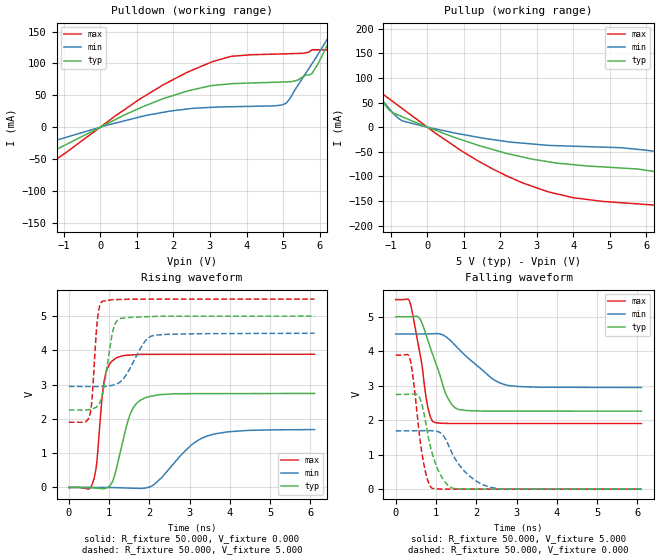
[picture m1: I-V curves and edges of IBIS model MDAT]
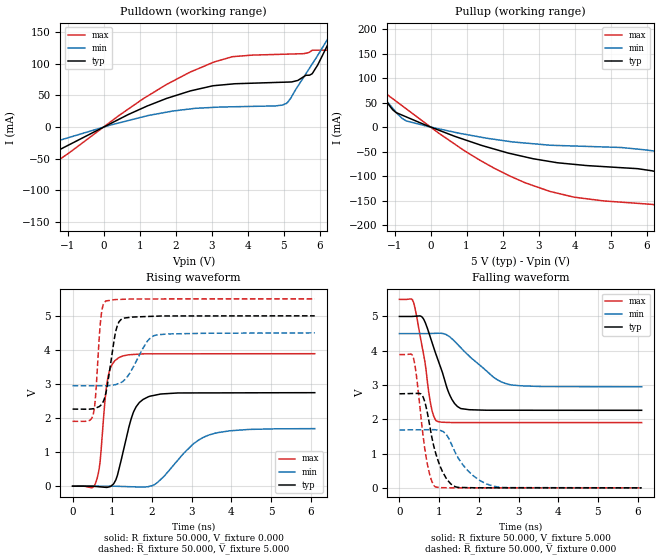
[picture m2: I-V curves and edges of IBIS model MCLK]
|Texas Instruments Incorporated
|1-Bit, 10MHz, 2nd-Order, Isolated Delta-Sigma Modulator
| Marketing part#  Voltage Range   Package-type   #pins
|AMC1203BDUB   4.5 to 5.5   SO-8, Gull-Wing   8
|AMC1203BDUBG4   4.5 to 5.5   SO-8, Gull-Wing   8
|AMC1203BDUBR   4.5 to 5.5   SO-8, Gull-Wing   8
|AMC1203BDUBRG4   4.5 to 5.5   SO-8, Gull-Wing   8
|AMC1203DUB   4.5 to 5.5   SO-8, Gull-Wing   8
|AMC1203DUBG4   4.5 to 5.5   SO-8, Gull-Wing   8
|AMC1203DUBR   4.5 to 5.5   SO-8, Gull-Wing   8
|AMC1203DUBRG4   4.5 to 5.5   SO-8, Gull-Wing   8
|AMC1203BDW   4.5 to 5.5   SO-16   16
|AMC1203BDWR   4.5 to 5.5   SO-16   16
|AMC1203DW   4.5 to 5.5   SO-16   16
|AMC1203DWR   4.5 to 5.5   SO-16   16
|AMC1203BPSA   4.5 to 5.5   SO-8   8
|AMC1203BPSAR   4.5 to 5.5   SO-8   8
|AMC1203PSA   4.5 to 5.5   SO-8   8
|AMC1203PSAR   4.5 to 5.5   SO-8   8
[IBIS Ver]   4.0
[File name]   amc1203.ibs
[File Rev]   1.0
[Date]   05/062010
[Source]   Texas Instruments Incorporated.
   Analog-eLab, HPA
   12500 TI Blvd
   Dallas, TX -75243
   For Support e-mail: elab_ibis@list.ti.com
[Notes]   Revision History:
   1.0: 05/062010
   - Initial version of the model
   - Initial Model generated from simulations in TISPICED
   - Specified temperature range = -40C to 105C. Device power
   dissipation is 110mW. Maximum theta jc (SO-8) = 164 C/W. IBIS
   test maximum temperature = 125C
   - Model not matched to measurements
   - Ignore warnings related to min and max values of ccomp,
   The device process of this product is CMOS. The ccomp
   values are based on PVT variations as seen in simulations
[Disclaimer]
 This product is designed as an aid for customers of Texas Instruments.
 No warranties, either expressed or implied, with respect to this third
 party software (if any) or with respect to its fitness for any
 particular purpose is claimed by Texas Instruments or the author. The
 software (if any) is provided solely on an "as is" basis. The entire
 risk as to its quality and performance is with the customer
[Copyright] (C) Copyright 2009 Texas Instruments Incorporated.
   All rights reserved.
|   AMC1203DUB - SO-8, Gull-Wing
[Component]   amc1203dub   |SO-8, Gull-Wing
[Manufacturer] TI
[Package]
| variable   typ   min   max
R_pkg  0.067958   0.033850   0.110020
L_pkg  4.035955nH  3.604460nH  4.524820nH
C_pkg  1.196889pF  1.079930pF  1.255480pF
[Pin] signal_name  model_name  R_pin  L_pin C_pin
1   VDD1   TERM   0.04382  4.49301nH  1.20573pF
2   VINP   TERM   0.08107  3.84004nH  1.21759pF
3   VINN   TERM   0.11002  4.52482nH  1.24194pF
4   GND1   TERM   0.03385  3.60446nH  1.12112pF
5   GND2   GND   0.04658  3.76318nH  1.07993pF
6   MDAT   MDAT   0.10060  4.30773nH  1.23091pF
7   MCLK   MCLK   0.08948  4.04013nH  1.22241pF
8   VDD2   POWER   0.03824  3.71427nH  1.25548pF
|   AMC1203PSA - SO-8
[Component]   amc1203pas   |SO-8
[Manufacturer] TI
[Package]
| variable   typ   min   max
R_pkg  0.082216   0.044190   0.126530
L_pkg  1.772578nH  1.469600nH  2.372740nH
C_pkg  0.346504pF  0.239380pF  0.477210pF
[Pin] signal_name  model_name  R_pin  L_pin C_pin
1   VDD1   TERM   0.06196  2.37274nH  0.46610pF
2   VINP   TERM   0.10341  1.72833nH  0.31281pF
3   VINN   TERM   0.12653  1.86934nH  0.25026pF
4   GND1   TERM   0.05629  2.10297nH  0.42922pF
5   GND2   GND   0.06651  1.50308nH  0.29801pF
6   MDAT   MDAT   0.11287  1.66363nH  0.23938pF
7   MCLK   MCLK   0.08597  1.47093nH  0.29904pF
8   VDD2   POWER   0.04419  1.46960nH  0.47721pF
|   AMC1203DW - SO-16
[Component]   amc1203dw   |SO-16
[Manufacturer] TI
[Package]
| variable   typ   min   max
R_pkg  0.038526   0.003610   0.111860
L_pkg  2.946539nH  1.634270nH  4.703810nH
C_pkg  0.921273pF  0.675660pF  1.374930pF
[Pin] signal_name  model_name  R_pin  L_pin C_pin
1   VDD1   TERM   0.04296  4.66236nH  1.26722pF
2   VINP   TERM   0.11186  4.70381nH  1.06049pF
3   VINN   TERM   0.09034  3.30153nH  0.76963pF
4   GND1   TERM   0.00361  1.63447nH  0.70855pF
5   NC   NC   0.00361  1.63427nH  0.70856pF
6   NC   NC   0.00370  1.66394nH  0.68405pF
7   NC   NC   0.00367  1.67094nH  0.67566pF
8   GND1   TERM   0.02804  4.12835nH  1.37395pF
9   GND2   GND   0.03564  4.05816nH  1.37493pF
10   NC   NC   0.09603  3.43032nH  0.78630pF
11   MDAT   MDAT   0.05441  2.62155nH  0.89494pF
12   NC   NC   0.00361  1.63430nH  0.70851pF
13   MCLK   MCLK   0.07390  2.89307nH  0.78596pF
14   VDD2   POWER   0.05191  3.03712nH  0.82076pF
15   NC   NC   0.00565  2.62355nH  0.94964pF
16   GND2   GND   0.00747  3.44688nH  1.17122pF
|   TERM Model
[Model] TERM
Model_type Terminator
C_comp   1e-200   1e-200   1e-200
| variable   typ   min   max
[Voltage Range]   5.0V   4.5V   5.5V
[POWER Clamp Reference]  5.0V   4.5V   5.5V
[GND Clamp Reference]   0.0V   0.0V   0.0V
|Operating Temperature
[Temperature Range]   27   123   -40
| Models and submodels in the file (3): TERM (Terminator), MDAT (Output), MCLK (Output)
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|   MDAT Model
[Model] MDAT
Model_type Output
Polarity   Non-Inverting
Enable   Active-Low
Vmeas = 2.5
Vref = 2.5
Cref = 15pF
Rref = 50
|   typ   min   max
|   MDAT HIGH
C_comp   1.446901E-12   1.464566E-12   1.435600E-012
|   MDAT LOW
|C_comp   3.656083E-13   3.837180E-13   2.354078E-13
|   average
|C_comp   9.062547E-13   7.178000E-02   9.241420E-13
| variable   typ   min   max
[Voltage Range]   5   4.5   5.5
[Temperature Range]   27   125   -40
[Pullup Reference]   5   4.5   5.5
[Pulldown Reference]   0   0   0
[Power Clamp Reference]   5   4.5   5.5
[GND Clamp Reference]   0   0   0
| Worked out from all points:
|   slope of the pulldown table from 0 to 0.75 V, typ, clamps not added: 34.8 ohm
|   slope of the pullup table from 0 to 0.75 V, typ, clamps not added: 35.6 ohm
|   falling waveform, R_fixture 50.000, V_fixture 5.000: 20-80 % time 469ps typ, 877ps min, 292ps max; typ from 5 V to 2.26 V
|   rising waveform, R_fixture 50.000, V_fixture 0.000: 20-80 % time 363ps typ, 832ps min, 180ps max; typ from 0 V to 2.74 V
|   rising waveform, R_fixture 50.000, V_fixture 5.000: 20-80 % time 219ps typ, 442ps min, 122ps max; typ from 2.26 V to 5 V
|   falling waveform, R_fixture 50.000, V_fixture 0.000: 20-80 % time 353ps typ, 595ps min, 245ps max; typ from 2.74 V to 0 V
[Pulldown]
|   Voltage   I(typ)   I(min)   I(max)
-5V       -138.1mA   -85.42mA   -187.7mA
-3.408V   -95.74mA   -58.23mA   -133.2mA
-1.909V   -55.62mA   -32.63mA   -78.2mA
1.207V    33.19mA    17.88mA    48.53mA
3.065V    65.4mA     31.15mA    102.8mA
3.59V     68.14mA    32.05mA    111.2mA
5.074V    71mA       37.3mA     115.2mA
5.798V    84.8mA     100.1mA    121.4mA
6.271V    135.5mA    143.7mA    121.4mA
6.444V    156.6mA    159.8mA    129.9mA
6.765V    196mA      189.8mA    179mA
9.985V    614.1mA    504.7mA    747.7mA
[Pullup]
|   Voltage   I(typ)   I(min)   I(max)
-5V       522.2mA    410.7mA    693.7mA
-1.677V   107.2mA    95.67mA    130.1mA
-1.302V   62.26mA    60.51mA    73.91mA
-1.049V   35.22mA    38.3mA     57.8mA
-671.2mV  20.68mA    12.62mA    37.04mA
965.9mV   -26.22mA   -14.87mA   -49.49mA
2.648V    -61.31mA   -32.74mA   -114.3mA
4.002V    -76.27mA   -38.71mA   -143.3mA
5.758V    -85.05mA   -45.07mA   -155.8mA
6.65V     -96.68mA   -53.55mA   -165.8mA
8.43V     -132.3mA   -77.87mA   -210.5mA
9.985V    -179mA     -109.2mA   -268.9mA
[Ramp]
R_load = 50
|   typ   min   max
dV/dt_r   1.64642/3.62454e-010   1.02817/8.2858e-010   2.33306/1.79539e-010
dV/dt_f   1.64308/4.68889e-010  0.931405/8.7379e-010   2.19199/2.91254e-010
[Falling Waveform]
R_fixture = 50.000
V_fixture = 5.000
V_fixture_min = 4.500
V_fixture_max = 5.500
C_fixture = 0.000
|  time   V(typ)   V(min)   V(max)
0s        5V         4.5V       5.498V
360.1ps   5.003V     4.5V       5.391V
611.2ps   4.918V     4.5V       3.878V
794.7ps   4.336V     4.504V     2.396V
941.1ps   3.829V     4.509V     1.948V
1.269ns   2.703V     4.404V     1.907V
1.552ns   2.312V     4.082V     1.904V
2.377ns   2.264V     3.222V     1.904V
2.775ns   2.264V     3.012V     1.904V
6.102ns   2.262V     2.948V     1.903V
[Rising Waveform]
R_fixture = 50.000
V_fixture = 0.000
V_fixture_min = 0.000
V_fixture_max = 0.000
C_fixture = 0.000
|  time   V(typ)   V(min)   V(max)
0s        34.01nV    678.5uV    15.45nV
588.2ps   -9.442mV   686.6uV    115.5mV
692.8ps   -20.18mV   688uV      707.2mV
818.3ps   -33.07mV   689.8uV    2.525V
888ps     -30.59mV   690.7uV    3.174V
1.165ns   480.4mV    -5.795mV   3.771V
1.527ns   2.152V     -19.22mV   3.865V
1.909ns   2.624V     -13.95mV   3.884V
3.429ns   2.738V     1.499V     3.886V
6.102ns   2.744V     1.689V     3.888V
[Rising Waveform]
R_fixture = 50.000
V_fixture = 5.000
V_fixture_min = 4.500
V_fixture_max = 5.500
C_fixture = 0.000
|  time   V(typ)   V(min)   V(max)
0s        2.262V     2.948V     1.903V
520.6ps   2.272V     2.946V     2.107V
583.3ps   2.292V     2.946V     2.701V
713.2ps   2.379V     2.945V     4.931V
837.1ps   2.719V     2.945V     5.435V
1.094ns   4.575V     2.984V     5.478V
1.274ns   4.927V     3.08V      5.486V
1.883ns   4.981V     4.253V     5.496V
2.111ns   4.99V      4.438V     5.496V
6.102ns   5V         4.5V       5.498V
[Falling Waveform]
R_fixture = 50.000
V_fixture = 0.000
V_fixture_min = 0.000
V_fixture_max = 0.000
C_fixture = 0.000
|  time   V(typ)   V(min)   V(max)
0s        2.744V     1.689V     3.888V
351.3ps   2.753V     1.692V     3.792V
566.3ps   2.707V     1.694V     1.808V
677.6ps   2.329V     1.695V     859.1mV
903.9ps   1.051V     1.694V     27.05mV
1.18ns    275.3mV    1.558V     2.803mV
1.405ns   33.53mV    1.033V     645.7uV
1.858ns   2.999mV    354.3mV    583.5uV
2.367ns   1.442mV    49.27mV    513.5uV
6.102ns   41.19nV    678.5uV    17.93nV
|   MCLK Model
[Model] MCLK
Model_type Output
Polarity   Non-Inverting
Enable   Active-Low
Vmeas = 2.5
Vref = 2.5
Cref = 15pF
Rref = 50
|   typ   min   max
|   MCLK HIGH
C_comp   1.446533E-12   1.462987E-12   1.435514E-12
|   MCLK LOW
|C_comp   3.668114E-13   3.922605E-13   2.384701E-13
|   average
|C_comp   9.066722E-13   9.276238E-13   8.369921E-13
| variable   typ   min   max
[Voltage Range]   5   4.5   5.5
[Temperature Range]   27   125   -40
[Pullup Reference]   5   4.5   5.5
[Pulldown Reference]   0   0   0
[Power Clamp Reference]   5   4.5   5.5
[GND Clamp Reference]   0   0   0
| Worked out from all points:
|   slope of the pulldown table from 0 to 0.75 V, typ, clamps not added: 34.8 ohm
|   slope of the pullup table from 0 to 0.75 V, typ, clamps not added: 35.6 ohm
|   falling waveform, R_fixture 50.000, V_fixture 5.000: 20-80 % time 469ps typ, 877ps min, 292ps max; typ from 5 V to 2.26 V
|   rising waveform, R_fixture 50.000, V_fixture 0.000: 20-80 % time 363ps typ, 832ps min, 180ps max; typ from 0 V to 2.74 V
|   rising waveform, R_fixture 50.000, V_fixture 5.000: 20-80 % time 219ps typ, 442ps min, 122ps max; typ from 2.26 V to 5 V
|   falling waveform, R_fixture 50.000, V_fixture 0.000: 20-80 % time 353ps typ, 595ps min, 245ps max; typ from 2.74 V to 0 V
[Pulldown]
|   Voltage   I(typ)   I(min)   I(max)
-5V       -138.1mA   -85.42mA   -187.7mA
-3.408V   -95.74mA   -58.23mA   -133.2mA
-1.909V   -55.62mA   -32.63mA   -78.2mA
1.207V    33.19mA    17.88mA    48.53mA
3.065V    65.4mA     31.15mA    102.8mA
3.59V     68.14mA    32.05mA    111.2mA
5.074V    71mA       37.3mA     115.2mA
5.798V    84.8mA     100.1mA    121.4mA
6.271V    135.5mA    143.7mA    121.4mA
6.444V    156.6mA    159.8mA    129.9mA
6.765V    196mA      189.8mA    179mA
9.985V    614.1mA    504.7mA    747.7mA
[Pullup]
|   Voltage   I(typ)   I(min)   I(max)
-5V       522.2mA    410.7mA    693.7mA
-1.677V   107.2mA    95.67mA    130.1mA
-1.302V   62.26mA    60.51mA    73.91mA
-1.049V   35.22mA    38.3mA     57.8mA
-671.2mV  20.68mA    12.62mA    37.04mA
965.9mV   -26.22mA   -14.87mA   -49.49mA
2.648V    -61.31mA   -32.74mA   -114.3mA
4.002V    -76.27mA   -38.71mA   -143.3mA
5.758V    -85.05mA   -45.07mA   -155.8mA
6.65V     -96.68mA   -53.55mA   -165.8mA
8.43V     -132.3mA   -77.87mA   -210.5mA
9.985V    -179mA     -109.2mA   -268.9mA
[Ramp]
R_load = 50
|   typ   min   max
dV/dt_r   1.64642/3.62454e-010   1.02817/8.2858e-010   2.33306/1.79539e-010
dV/dt_f   1.64308/4.68889e-010  0.931405/8.7379e-010   2.19199/2.91254e-010
[Falling Waveform]
R_fixture = 50.000
V_fixture = 5.000
V_fixture_min = 4.500
V_fixture_max = 5.500
C_fixture = 0.000
|  time   V(typ)   V(min)   V(max)
0s        5V         4.5V       5.498V
360.1ps   5.003V     4.5V       5.391V
611.2ps   4.918V     4.5V       3.878V
794.7ps   4.336V     4.504V     2.396V
941.1ps   3.829V     4.509V     1.948V
1.269ns   2.703V     4.404V     1.907V
1.552ns   2.312V     4.082V     1.904V
2.377ns   2.264V     3.222V     1.904V
2.775ns   2.264V     3.012V     1.904V
6.102ns   2.262V     2.948V     1.903V
[Rising Waveform]
R_fixture = 50.000
V_fixture = 0.000
V_fixture_min = 0.000
V_fixture_max = 0.000
C_fixture = 0.000
|  time   V(typ)   V(min)   V(max)
0s        34.01nV    678.5uV    15.45nV
588.2ps   -9.442mV   686.6uV    115.5mV
692.8ps   -20.18mV   688uV      707.2mV
818.3ps   -33.07mV   689.8uV    2.525V
888ps     -30.59mV   690.7uV    3.174V
1.165ns   480.4mV    -5.795mV   3.771V
1.527ns   2.152V     -19.22mV   3.865V
1.909ns   2.624V     -13.95mV   3.884V
3.429ns   2.738V     1.499V     3.886V
6.102ns   2.744V     1.689V     3.888V
[Rising Waveform]
R_fixture = 50.000
V_fixture = 5.000
V_fixture_min = 4.500
V_fixture_max = 5.500
C_fixture = 0.000
|  time   V(typ)   V(min)   V(max)
0s        2.262V     2.948V     1.903V
520.6ps   2.272V     2.946V     2.107V
583.3ps   2.292V     2.946V     2.701V
713.2ps   2.379V     2.945V     4.931V
837.1ps   2.719V     2.945V     5.435V
1.094ns   4.575V     2.984V     5.478V
1.274ns   4.927V     3.08V      5.486V
1.883ns   4.981V     4.253V     5.496V
2.111ns   4.99V      4.438V     5.496V
6.102ns   5V         4.5V       5.498V
[Falling Waveform]
R_fixture = 50.000
V_fixture = 0.000
V_fixture_min = 0.000
V_fixture_max = 0.000
C_fixture = 0.000
|  time   V(typ)   V(min)   V(max)
0s        2.744V     1.689V     3.888V
351.3ps   2.753V     1.692V     3.792V
566.3ps   2.707V     1.694V     1.808V
677.6ps   2.329V     1.695V     859.1mV
903.9ps   1.051V     1.694V     27.05mV
1.18ns    275.3mV    1.558V     2.803mV
1.405ns   33.53mV    1.033V     645.7uV
1.858ns   2.999mV    354.3mV    583.5uV
2.367ns   1.442mV    49.27mV    513.5uV
6.102ns   41.19nV    678.5uV    17.93nV
